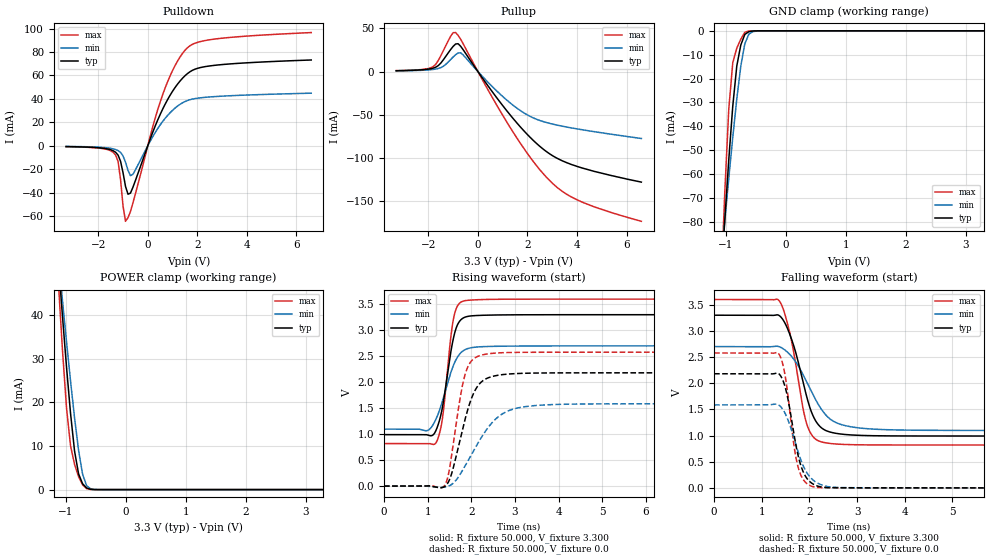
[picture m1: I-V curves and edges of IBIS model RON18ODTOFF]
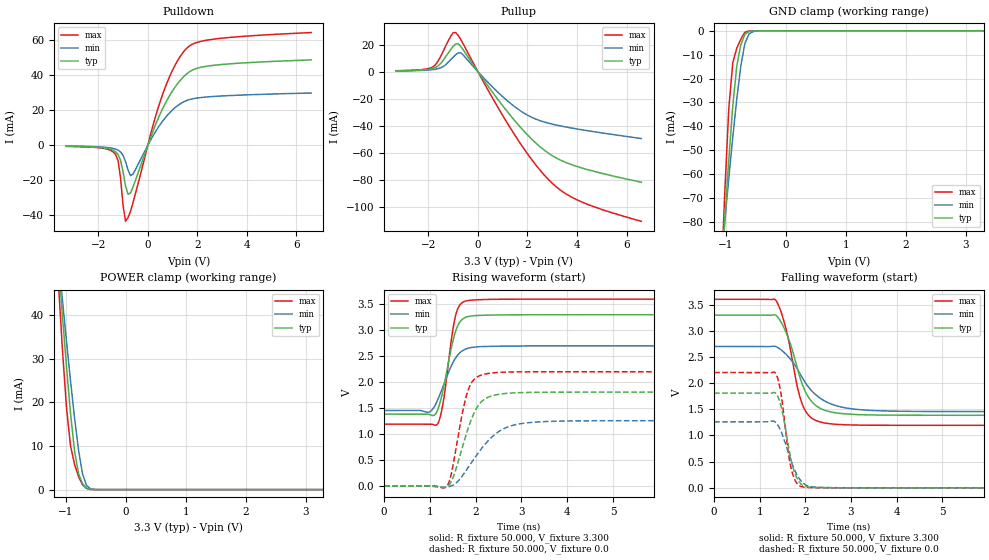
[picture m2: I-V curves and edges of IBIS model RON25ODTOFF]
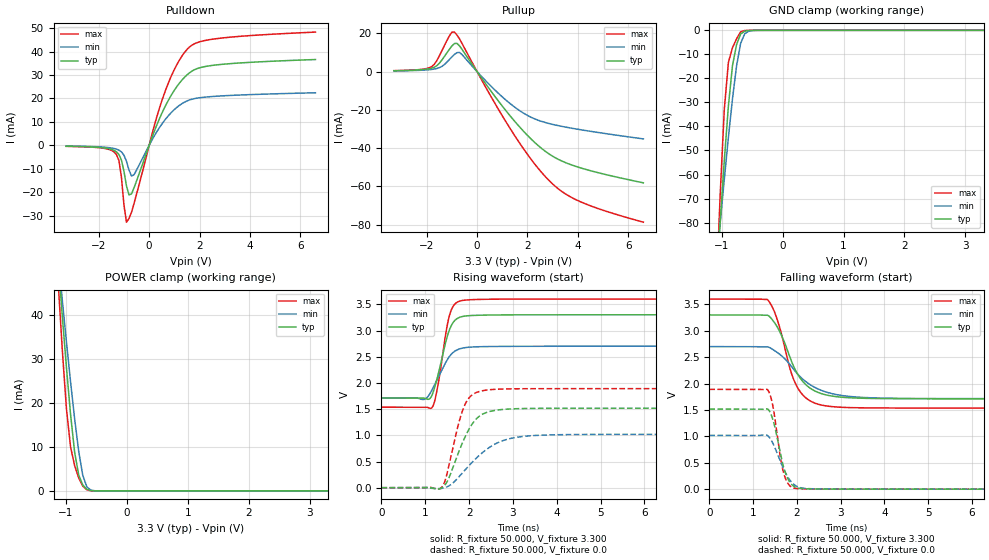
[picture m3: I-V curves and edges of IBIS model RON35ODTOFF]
| This IBIS file was created by s2ibis3 version 1.1
| North Carolina State University, ERL, 2006
[IBIS ver] 5.0
[File name] s34ml02g3_b_i_33_r1.ibs
[File Rev] 1.0
| Rev1.0 Initial release (ONFI)
[Date] 1/21/2022
[Source] Cypress IBIS team
|   Email: dl.ibisteam@cypress.com
[Notes]  Generated IBIS models from SPICE simulations.
|   VIO=3.3V, Temperature Range: Industrial (-40oC to +85oC).
[Disclaimer] THE MODEL LIBRARIES ARE PROVIDED AS IS.
[Copyright] (C) COPYRIGHT 2022
| CYPRESS SEMICONDUCTOR(An Infineon Technologies Company)
| ALL RIGHTS RESERVED.
|   Component S34ML02G3 SLC NAND in VBM063 package
[Component] S34ML02G3
[Manufacturer] Cypress
[Package]
| variable   typ   min   max
R_pkg   0.23446   0.1409   0.39955
L_pkg   4.678e-9   2.048e-9   8.953e-9
C_pkg   8.785e-13   4.724e-13   1.611e-12
[Pin]   signal_name   model_name   R_pin   L_pin   C_pin
A1   R   NC
A2   R   NC
A9   R   NC
A10   R   NC
B1   R   NC
B9   R   NC
B10   R   NC
C3   WP#   INPUT   0.32362   6.966E-09   1.196E-12
C4   ALE   INPUT   0.28665   6.74E-09   1.054E-12
C5   VSS   GND
C6   CE#   INPUT   0.32543   7.21E-09   1.01E-12
C7   WE#   INPUT   0.39955   8.95E-09   1.61E-12
C8   RB#   INPUT   0.29758   6.49E-09   9.88E-13
D3   VCC   NC
D4   RE#   INPUT   0.34398   7.76E-09   1.43E-12
D5   CLE   INPUT   0.28793   6.42E-09   9.82E-13
D6   R   NC
D7   R   NC
D8   R   NC
E3   R   NC
E4   R   NC
E5   R   NC
E6   R   NC
E7   R   NC
E8   R   NC
F3   R   NC
F4   R   NC
F5   R   NC
F6   R   NC
F7   VSS   NC
F8   R   NC
G3   R   NC
G4   VCC   NC
G5   VPE   INPUT   0.20739   3.83E-09   8.89E-13
G6   R   NC
G7   R   NC
G8   R   NC
H3   R   NC
H4   I/O0   N_IO   0.18604   3.52E-09   4.72E-13
H5   R   NC
H6   R   NC
H7   R   NC
H8   VCC   POWER
J3   R   NC
J4   I/O1   N_IO   0.16898   2.87E-09   5.43E-13
J5   R   NC
J6   VCC   POWER
J7   I/O5   N_IO   0.16649   2.56E-09   5.21E-13
J8   I/O7   N_IO   0.17054   2.57E-09   5.27E-13
K3   VSS   GND
K4   I/O2   N_IO   0.16236   2.71E-09   7.30E-13
K5   I/O3   N_IO   0.14284   2.05E-09   7.06E-13
K6   I/O4   N_IO   0.1409   2.12E-09   6.75E-13
K7   I/O6   N_IO   0.14112   2.09E-09   7.26E-13
K8   VSS   GND
L1   R   NC
L2   R   NC
L9   R   NC
L10   R   NC
M1   R   NC
M2   R   NC
M9   R   NC
M10   R   NC
[Model Selector] N_IO
RON18ODTOFF RON18ODTOFF
RON25ODTOFF RON25ODTOFF
RON35ODTOFF RON35ODTOFF
RON50ODTOFF RON50ODTOFF
| Models and submodels in the file (5): RON18ODTOFF (I/O), RON25ODTOFF (I/O), RON35ODTOFF (I/O), RON50ODTOFF (I/O), INPUT (Input)
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|   Model RON18ODTOFF
[Model] RON18ODTOFF
Model_type I/O
Polarity   Non-Inverting
Enable   Active-High
Vinl =  0.660V
Vinh =  2.640V
Vmeas =  1.650V
Cref =  2.000pF
Rref =  50.000
Vref =  1.650V
C_comp   2.860pF   2.840pF   2.890pF
[Model Spec]
Vinh   2.640V   2.160V   2.880V
Vinl   0.660V   0.540V   0.720V
Vmeas   1.650V   1.350V   1.800V
Vref   1.650V   1.350V   1.800V
Cref   2.000pF   NA   NA
Rref   50.000   NA   NA
[Temperature Range]   25.000   85.000   -40.000
[Voltage Range]   3.300V   2.700V   3.600V
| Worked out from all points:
|   slope of the pulldown table from 0 to 0.495 V, typ, clamps not added: 18.7 ohm
|   slope of the pullup table from 0 to 0.495 V, typ, clamps not added: 24.7 ohm
|   GND clamp passes 1 mA (typ) near -0.66 V on its own axis
|   POWER clamp passes 1 mA (typ) near -0.70 V on its own axis
|   rising waveform, R_fixture 50.000, V_fixture 3.300: 20-80 % time 264ps typ, 365ps min, 207ps max; typ from 0.991 V to 3.3 V
|   rising waveform, R_fixture 50.000, V_fixture 0.0: 20-80 % time 418ps typ, 721ps min, 295ps max; typ from 0 V to 2.18 V
|   falling waveform, R_fixture 50.000, V_fixture 3.300: 20-80 % time 415ps typ, 587ps min, 333ps max; typ from 3.3 V to 0.991 V
|   falling waveform, R_fixture 50.000, V_fixture 0.0: 20-80 % time 277ps typ, 365ps min, 226ps max; typ from 2.18 V to 0 V
[Pulldown]
|Voltage   I(typ)   I(min)   I(max)
-3.3V     -755uA     -586.6uA   -825.8uA
-1.3V     -5.583mA   -3.239mA   -7.938mA
-1.2V     -8.039mA   -4.15mA    -13.48mA
-1V       -23.07mA   -8.674mA   -51.47mA
-900mV    -34.68mA   -14.06mA   -64.49mA
-800mV    -41.4mA    -20.94mA   -61.39mA
-600mV    -35.44mA   -24.39mA   -48.81mA
600mV     31.2mA     20.64mA    43.51mA
1.1V      49.63mA    32.11mA    68.37mA
1.6V      61.51mA    38.57mA    83.57mA
2.8V      68.83mA    42.04mA    91.26mA
6.6V      73.15mA    44.83mA    96.55mA
[Pullup]
|Voltage   I(typ)   I(min)   I(max)
-3.3V     991.4uA    777.9uA    1.069mA
-1.8V     4.029mA    2.501mA    5.889mA
-1.5V     9.785mA    4.543mA    18.25mA
-1.1V     25.54mA    13.97mA    40.87mA
-900mV    31.89mA    19.52mA    45.09mA
-600mV    25.4mA     19.38mA    32.34mA
1.3V      -50.07mA   -36.2mA    -64.55mA
2V        -72.86mA   -50.16mA   -94.73mA
2.8V      -93.2mA    -59.17mA   -123.2mA
3.4V      -103.1mA   -63.11mA   -138.3mA
4V        -109.6mA   -66.26mA   -148.2mA
6.6V      -127.8mA   -77.36mA   -173.1mA
[GND_clamp]
|Voltage   I(typ)   I(min)   I(max)
-3.3V     -1.091A    -761mA     -1.739A
-1.089V   -106.4mA   -98.63mA   -110mA
-1.022V   -79.54mA   -80.06mA   -68.12mA
-955mV    -54.15mA   -61.98mA   -32.91mA
-888mV    -31.54mA   -44.64mA   -13.37mA
-821mV    -14.71mA   -28.56mA   -7.248mA
-754mV    -5.951mA   -14.81mA   -3.53mA
-687mV    -1.508mA   -5.409mA   -606.1uA
-620mV    -369.5uA   -1.421mA   -79.63uA
-553mV    -79.73uA   -350.6uA   -8.879uA
-486mV    -14.59uA   -85.42uA   -793.1nA
3.3V      0A         0A         0A
[POWER_clamp]
|Voltage   I(typ)   I(min)   I(max)
-3.3V     484mA      387mA      621.1mA
-1.122V   51.69mA    52.79mA    47mA
-1.055V   39.6mA     43.22mA    31.83mA
-988mV    28.05mA    33.88mA    18.67mA
-921mV    17.46mA    24.87mA    10.02mA
-854mV    8.817mA    16.42mA    5.78mA
-787mV    3.61mA     8.999mA    2.955mA
-720mV    1.342mA    3.534mA    1.088mA
-653mV    380.8uA    901.7uA    235uA
-586mV    72.64uA    176uA      28.35uA
-452mV    1.393uA    5.4uA      201.2nA
3.3V      0A         0A         3.891nA
[Ramp]
| variable   typ   min   max
dV/dt_r   1.309/0.419n   0.951/0.722n   1.547/0.296n
dV/dt_f   1.385/0.416n   0.962/0.588n   1.669/0.333n
R_load = 50.000
| The next line is not an IBIS keyword
| [Initial Delay]   1.100ns   1.900ns   0.430ns
[Rising Waveform]
R_fixture= 50.000
V_fixture= 3.300
V_fixture_min= 2.700
V_fixture_max= 3.600
|time   V(typ)   V(min)   V(max)
0s        991mV      1.097V     819.1mV
982ps     988mV      1.068V     819.7mV
1.112ns   977.5mV    1.164V     804.4mV
1.206ns   1.1V       1.315V     853.2mV
1.343ns   1.532V     1.646V     1.318V
1.515ns   2.496V     2.141V     2.745V
1.599ns   2.875V     2.339V     3.247V
1.699ns   3.129V     2.503V     3.489V
1.869ns   3.256V     2.632V     3.572V
19.57ns   3.3V       2.7V       3.6V
[Rising Waveform]
R_fixture= 50.000
V_fixture= 0.0
V_fixture_min= 0.0
V_fixture_max= 0.0
|time   V(typ)   V(min)   V(max)
0s        -5.427nV   -1.386uV   5.918nV
1.386ns   -10.79mV   -19.76mV   7.575mV
1.544ns   220.6mV    28.07mV    556.3mV
1.743ns   892.6mV    224.8mV    1.685V
1.874ns   1.335V     410.4mV    2.19V
2.096ns   1.857V     744.4mV    2.475V
2.353ns   2.072V     1.09V      2.543V
2.88ns    2.16V      1.46V      2.573V
3.91ns    2.18V      1.571V     2.578V
19.57ns   2.181V     1.585V     2.578V
[Falling Waveform]
R_fixture= 50.000
V_fixture= 3.300
V_fixture_min= 2.700
V_fixture_max= 3.600
|time   V(typ)   V(min)   V(max)
0s        3.3V       2.7V       3.6V
1.364ns   3.295V     2.698V     3.578V
1.599ns   2.909V     2.541V     2.921V
1.859ns   2.054V     2.177V     1.553V
1.949ns   1.723V     2.012V     1.208V
2.129ns   1.284V     1.688V     931.5mV
2.37ns    1.086V     1.369V     856.5mV
2.829ns   1.014V     1.174V     826.7mV
3.899ns   992.3mV    1.106V     819.4mV
19.57ns   991mV      1.097V     819.1mV
[Falling Waveform]
R_fixture= 50.000
V_fixture= 0.0
V_fixture_min= 0.0
V_fixture_max= 0.0
|time   V(typ)   V(min)   V(max)
0s        2.181V     1.585V     2.578V
1.353ns   2.184V     1.585V     2.568V
1.426ns   2.092V     1.52V      2.417V
1.486ns   1.944V     1.432V     2.169V
1.677ns   1.023V     948.7mV    803.1mV
1.768ns   598mV      674mV      380mV
1.922ns   215mV      328.1mV    102.1mV
2.133ns   47.14mV    110.9mV    10.97mV
2.923ns   1.063mV    2.608mV    441uV
19.57ns   4.386nV    7.005nV    5.61nV
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|   Model RON25ODTOFF
[Model] RON25ODTOFF
Model_type I/O
Polarity   Non-Inverting
Enable   Active-High
Vinl =  0.660V
Vinh =  2.640V
Vmeas =  1.650V
Cref =  2.000pF
Rref =  50.000
Vref =  1.650V
C_comp   2.860pF   2.840pF   2.890pF
[Model Spec]
Vinh   2.640V   2.160V   2.880V
Vinl   0.660V   0.540V   0.720V
Vmeas   1.650V   1.350V   1.800V
Vref   1.650V   1.350V   1.800V
Cref   2.000pF   NA   NA
Rref   50.000   NA   NA
[Temperature Range]   25.000   85.000   -40.000
[Voltage Range]   3.300V   2.700V   3.600V
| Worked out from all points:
|   slope of the pulldown table from 0 to 0.495 V, typ, clamps not added: 27.8 ohm
|   slope of the pullup table from 0 to 0.495 V, typ, clamps not added: 38.7 ohm
|   GND clamp passes 1 mA (typ) near -0.66 V on its own axis
|   POWER clamp passes 1 mA (typ) near -0.70 V on its own axis
|   rising waveform, R_fixture 50.000, V_fixture 3.300: 20-80 % time 272ps typ, 358ps min, 220ps max; typ from 1.39 V to 3.3 V
|   rising waveform, R_fixture 50.000, V_fixture 0.0: 20-80 % time 405ps typ, 683ps min, 290ps max; typ from 0 V to 1.81 V
|   falling waveform, R_fixture 50.000, V_fixture 3.300: 20-80 % time 441ps typ, 656ps min, 350ps max; typ from 3.3 V to 1.39 V
|   falling waveform, R_fixture 50.000, V_fixture 0.0: 20-80 % time 241ps typ, 314ps min, 199ps max; typ from 1.81 V to 0 V
[Pulldown]
|Voltage   I(typ)   I(min)   I(max)
-3.3V     -502.5uA   -390.8uA   -549.8uA
-1.3V     -3.668mA   -2.141mA   -5.21mA
-1.2V     -5.254mA   -2.737mA   -8.768mA
-1.1V     -8.628mA   -3.751mA   -18.65mA
-900mV    -23.09mA   -9.22mA    -43.32mA
-800mV    -27.88mA   -13.96mA   -41.25mA
-600mV    -23.88mA   -16.46mA   -32.78mA
600mV     20.96mA    13.86mA    29.17mA
1.1V      33.25mA    21.51mA    45.74mA
1.6V      41.12mA    25.76mA    55.8mA
2.8V      45.9mA     28.04mA    60.85mA
6.6V      48.77mA    29.89mA    64.37mA
[Pullup]
|Voltage   I(typ)   I(min)   I(max)
-3.3V     629.8uA    494.3uA    679.1uA
-1.8V     2.541mA    1.582mA    3.707mA
-1.5V     6.13mA     2.86mA     11.5mA
-1.1V     16.26mA    8.853mA    26.06mA
-900mV    20.39mA    12.47mA    28.8mA
-600mV    16.25mA    12.41mA    20.65mA
500mV     -12.92mA   -9.648mA   -16.53mA
1.4V      -34.21mA   -24.6mA    -44.09mA
2.1V      -48.39mA   -32.97mA   -62.96mA
2.9V      -60.69mA   -38.18mA   -80.4mA
4.1V      -70.39mA   -42.51mA   -95.21mA
6.6V      -81.41mA   -49.27mA   -110.2mA
[GND_clamp]
|Voltage   I(typ)   I(min)   I(max)
-3.3V     -1.091A    -761mA     -1.739A
-1.089V   -106.4mA   -98.63mA   -110mA
-1.022V   -79.54mA   -80.06mA   -68.12mA
-955mV    -54.15mA   -61.98mA   -32.91mA
-888mV    -31.54mA   -44.64mA   -13.37mA
-821mV    -14.71mA   -28.56mA   -7.248mA
-754mV    -5.951mA   -14.81mA   -3.53mA
-687mV    -1.508mA   -5.409mA   -606.1uA
-620mV    -369.5uA   -1.421mA   -79.63uA
-553mV    -79.73uA   -350.6uA   -8.879uA
-486mV    -14.59uA   -85.42uA   -793.1nA
3.3V      0A         0A         0A
[POWER_clamp]
|Voltage   I(typ)   I(min)   I(max)
-3.3V     484mA      387mA      621.1mA
-1.122V   51.69mA    52.79mA    47mA
-1.055V   39.6mA     43.22mA    31.83mA
-988mV    28.05mA    33.88mA    18.67mA
-921mV    17.46mA    24.87mA    10.02mA
-854mV    8.817mA    16.42mA    5.78mA
-787mV    3.61mA     8.999mA    2.955mA
-720mV    1.342mA    3.534mA    1.088mA
-653mV    380.8uA    901.7uA    235uA
-586mV    72.64uA    176uA      28.35uA
-452mV    1.393uA    5.4uA      201.2nA
3.3V      0A         0A         3.891nA
[Ramp]
| variable   typ   min   max
dV/dt_r   1.086/0.406n   0.756/0.684n   1.321/0.290n
dV/dt_f   1.149/0.441n   0.746/0.655n   1.444/0.351n
R_load = 50.000
| The next line is not an IBIS keyword
| [Initial Delay]   1.100ns   1.900ns   0.430ns
[Rising Waveform]
R_fixture= 50.000
V_fixture= 3.300
V_fixture_min= 2.700
V_fixture_max= 3.600
|time   V(typ)   V(min)   V(max)
0s        1.386V     1.456V     1.194V
972ps     1.383V     1.422V     1.194V
1.093ns   1.364V     1.521V     1.178V
1.173ns   1.469V     1.663V     1.2V
1.297ns   1.878V     1.936V     1.636V
1.479ns   2.698V     2.332V     2.87V
1.569ns   2.995V     2.476V     3.304V
1.679ns   3.184V     2.585V     3.511V
1.855ns   3.268V     2.659V     3.575V
19.57ns   3.3V       2.7V       3.6V
[Rising Waveform]
R_fixture= 50.000
V_fixture= 0.0
V_fixture_min= 0.0
V_fixture_max= 0.0
|time   V(typ)   V(min)   V(max)
0s        -4.772nV   -1.614uV   8.052nV
1.369ns   -14.24mV   -19.23mV   -2.752mV
1.523ns   196.6mV    26.4mV     474mV
1.72ns    780.1mV    209mV      1.445V
1.849ns   1.145V     373.8mV    1.877V
2.058ns   1.551V     640.3mV    2.112V
2.322ns   1.728V     917.1mV    2.175V
2.828ns   1.794V     1.174V     2.198V
3.798ns   1.808V     1.25V      2.202V
19.57ns   1.809V     1.259V     2.202V
[Falling Waveform]
R_fixture= 50.000
V_fixture= 3.300
V_fixture_min= 2.700
V_fixture_max= 3.600
|time   V(typ)   V(min)   V(max)
0s        3.3V       2.7V       3.6V
1.345ns   3.298V     2.699V     3.588V
1.573ns   2.975V     2.554V     3.043V
1.823ns   2.283V     2.271V     1.931V
1.943ns   1.951V     2.086V     1.572V
2.167ns   1.62V      1.826V     1.315V
2.473ns   1.468V     1.635V     1.231V
3.064ns   1.402V     1.504V     1.2V
4.177ns   1.387V     1.461V     1.194V
19.57ns   1.386V     1.456V     1.194V
[Falling Waveform]
R_fixture= 50.000
V_fixture= 0.0
V_fixture_min= 0.0
V_fixture_max= 0.0
|time   V(typ)   V(min)   V(max)
0s        1.809V     1.259V     2.202V
1.344ns   1.812V     1.255V     2.192V
1.406ns   1.726V     1.186V     2.054V
1.462ns   1.575V     1.088V     1.82V
1.622ns   826.8mV    683.4mV    696.2mV
1.699ns   487.1mV    483.3mV    332.2mV
1.809ns   194.6mV    258.4mV    92.38mV
1.969ns   35.69mV    78.59mV    14.33mV
2.819ns   1.298mV    2.269mV    787.2uV
19.57ns   5.636nV    10.69nV    7.687nV
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|   Model RON35ODTOFF
[Model] RON35ODTOFF
Model_type I/O
Polarity   Non-Inverting
Enable   Active-High
Vinl =  0.660V
Vinh =  2.640V
Vmeas =  1.650V
Cref =  2.000pF
Rref =  50.000
Vref =  1.650V
C_comp   2.860pF   2.840pF   2.890pF
[Model Spec]
Vinh   2.640V   2.160V   2.880V
Vinl   0.660V   0.540V   0.720V
Vmeas   1.650V   1.350V   1.800V
Vref   1.650V   1.350V   1.800V
Cref   2.000pF   NA   NA
Rref   50.000   NA   NA
[Temperature Range]   25.000   85.000   -40.000
[Voltage Range]   3.300V   2.700V   3.600V
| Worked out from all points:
|   slope of the pulldown table from 0 to 0.495 V, typ, clamps not added: 36.8 ohm
|   slope of the pullup table from 0 to 0.495 V, typ, clamps not added: 53.9 ohm
|   GND clamp passes 1 mA (typ) near -0.66 V on its own axis
|   POWER clamp passes 1 mA (typ) near -0.70 V on its own axis
|   rising waveform, R_fixture 50.000, V_fixture 3.300: 20-80 % time 285ps typ, 370ps min, 235ps max; typ from 1.71 V to 3.3 V
|   rising waveform, R_fixture 50.000, V_fixture 0.0: 20-80 % time 474ps typ, 788ps min, 342ps max; typ from 0 V to 1.52 V
|   falling waveform, R_fixture 50.000, V_fixture 3.300: 20-80 % time 537ps typ, 768ps min, 437ps max; typ from 3.3 V to 1.71 V
|   falling waveform, R_fixture 50.000, V_fixture 0.0: 20-80 % time 254ps typ, 331ps min, 210ps max; typ from 1.52 V to 0 V
[Pulldown]
|Voltage   I(typ)   I(min)   I(max)
-3.3V     -376.3uA   -292.9uA   -411.8uA
-1.3V     -2.711mA   -1.593mA   -3.845mA
-1.2V     -3.862mA   -2.031mA   -6.412mA
-1.1V     -6.295mA   -2.773mA   -13.53mA
-900mV    -17.29mA   -6.801mA   -32.74mA
-800mV    -21.13mA   -10.47mA   -31.18mA
-600mV    -18.1mA    -12.5mA    -24.76mA
500mV     13.57mA    9.008mA    18.88mA
1V        23.5mA     15.27mA    32.34mA
1.5V      30.02mA    18.93mA    40.86mA
2.6V      34.2mA     20.9mA     45.38mA
6.6V      36.59mA    22.42mA    48.28mA
[Pullup]
|Voltage   I(typ)   I(min)   I(max)
-3.3V     449uA      352.5uA    484.2uA
-1.8V     1.797mA    1.122mA    2.616mA
-1.5V     4.303mA    2.018mA    8.121mA
-1.1V     11.63mA    6.293mA    18.65mA
-900mV    14.64mA    8.944mA    20.66mA
-600mV    11.67mA    8.93mA     14.81mA
500mV     -9.277mA   -6.933mA   -11.85mA
1.4V      -24.55mA   -17.66mA   -31.59mA
2.1V      -34.69mA   -23.62mA   -45.09mA
2.9V      -43.45mA   -27.31mA   -57.54mA
4.1V      -50.33mA   -30.39mA   -68.06mA
6.6V      -58.19mA   -35.22mA   -78.77mA
[GND_clamp]
|Voltage   I(typ)   I(min)   I(max)
-3.3V     -1.091A    -761mA     -1.739A
-1.089V   -106.4mA   -98.63mA   -110mA
-1.022V   -79.54mA   -80.06mA   -68.12mA
-955mV    -54.15mA   -61.98mA   -32.91mA
-888mV    -31.54mA   -44.64mA   -13.37mA
-821mV    -14.71mA   -28.56mA   -7.248mA
-754mV    -5.951mA   -14.81mA   -3.53mA
-687mV    -1.508mA   -5.409mA   -606.1uA
-620mV    -369.5uA   -1.421mA   -79.63uA
-553mV    -79.73uA   -350.6uA   -8.879uA
-486mV    -14.59uA   -85.42uA   -793.1nA
3.3V      0A         0A         0A
[POWER_clamp]
|Voltage   I(typ)   I(min)   I(max)
-3.3V     484mA      387mA      621.1mA
-1.122V   51.69mA    52.79mA    47mA
-1.055V   39.6mA     43.22mA    31.83mA
-988mV    28.05mA    33.88mA    18.67mA
-921mV    17.46mA    24.87mA    10.02mA
-854mV    8.817mA    16.42mA    5.78mA
-787mV    3.61mA     8.999mA    2.955mA
-720mV    1.342mA    3.534mA    1.088mA
-653mV    380.8uA    901.7uA    235uA
-586mV    72.64uA    176uA      28.35uA
-452mV    1.393uA    5.4uA      201.2nA
3.3V      0A         0A         3.891nA
[Ramp]
| variable   typ   min   max
dV/dt_r   0.910/0.475n   0.611/0.790n   1.134/0.342n
dV/dt_f   0.953/0.537n   0.592/0.767n   1.238/0.438n
R_load = 50.000
| The next line is not an IBIS keyword
| [Initial Delay]   1.100ns   1.900ns   0.430ns
[Rising Waveform]
R_fixture= 50.000
V_fixture= 3.300
V_fixture_min= 2.700
V_fixture_max= 3.600
|time   V(typ)   V(min)   V(max)
0s        1.712V     1.714V     1.536V
971ps     1.71V      1.684V     1.537V
1.083ns   1.689V     1.764V     1.523V
1.16ns    1.778V     1.877V     1.535V
1.277ns   2.105V     2.074V     1.899V
1.471ns   2.793V     2.397V     2.957V
1.56ns    3.03V      2.513V     3.31V
1.68ns    3.196V     2.608V     3.509V
1.88ns    3.273V     2.669V     3.577V
19.57ns   3.3V       2.7V       3.6V
[Rising Waveform]
R_fixture= 50.000
V_fixture= 0.0
V_fixture_min= 0.0
V_fixture_max= 0.0
|time   V(typ)   V(min)   V(max)
0s        -3.954nV   -1.708uV   9.825nV
1.36ns    -11.21mV   -15.11mV   -3.94mV
1.474ns   80.25mV    8.573mV    195.3mV
1.744ns   638.8mV    185.1mV    1.17V
1.914ns   979.2mV    343.9mV    1.6V
2.153ns   1.303V     554.6mV    1.812V
2.432ns   1.446V     750.7mV    1.867V
3.002ns   1.505V     949.9mV    1.887V
3.981ns   1.516V     1.011V     1.89V
19.57ns   1.517V     1.018V     1.89V
[Falling Waveform]
R_fixture= 50.000
V_fixture= 3.300
V_fixture_min= 2.700
V_fixture_max= 3.600
|time   V(typ)   V(min)   V(max)
0s        3.3V       2.7V       3.6V
1.334ns   3.293V     2.695V     3.585V
1.529ns   3.103V     2.602V     3.266V
1.649ns   2.91V      2.526V     2.936V
1.849ns   2.481V     2.352V     2.262V
2.014ns   2.182V     2.181V     1.924V
2.287ns   1.922V     1.987V     1.68V
2.707ns   1.778V     1.83V      1.572V
4.427ns   1.714V     1.718V     1.537V
19.57ns   1.712V     1.714V     1.536V
[Falling Waveform]
R_fixture= 50.000
V_fixture= 0.0
V_fixture_min= 0.0
V_fixture_max= 0.0
|time   V(typ)   V(min)   V(max)
0s        1.517V     1.018V     1.89V
1.334ns   1.516V     1.013V     1.879V
1.39ns    1.452V     960.1mV    1.779V
1.448ns   1.324V     874.2mV    1.588V
1.619ns   687.6mV    536.4mV    614.6mV
1.699ns   409.1mV    377.5mV    300.4mV
1.819ns   157.9mV    195.3mV    80.1mV
1.988ns   29.85mV    57.98mV    13.35mV
2.963ns   1.143mV    1.815mV    724.8uV
19.57ns   6.916nV    12.46nV    9.572nV
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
